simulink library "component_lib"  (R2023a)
settings: Solver=VariableStepAuto  StartTime=0.0  StopTime=10.0  RelTol=1e-3
undefined symbols (not defined in the file or in its folder): component_lib, ECCV_r, KoblenzTrier, mm, par, param_TD04, R1234yf_ph, SigIdentifier, Systems, TH0023_WP120, Thermal, V_nom
libraries: base_lib x166, $bdroot x164, simulink x2, slpidlib x1
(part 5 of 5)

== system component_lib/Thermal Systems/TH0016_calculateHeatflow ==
  "CL: (T1, p1, W1)" : Inport
  "CL: (T2, p2, W2)" : Inport  Port=2
  Constant2 : Constant  Value=par.cp_clt
  Demux : Demux  Outputs=3
  Demux1 : Demux  Outputs=3
  Product : Product  Inputs=3
  Sum : Sum  Inputs=|-+
  Terminator : Terminator
  Terminator1 : Terminator
  Terminator2 : Terminator
  Q [J/s] : Outport
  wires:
  "CL: (T1, p1, W1)"/1 -> Demux/1
  "CL: (T2, p2, W2)"/1 -> Demux1/1
  Constant2/1 -> Product/2
  Product/1 -> Q [J/s]/1
  Demux/2 -> Terminator/1
  Demux1/2 -> Terminator1/1
  Demux1/3 -> Terminator2/1
  Demux1/1 -> Sum/2
  Sum/1 -> Product/1
  Demux/1 -> Sum/1
  Demux/3 -> Product/3

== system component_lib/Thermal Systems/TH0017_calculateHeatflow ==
  "AIR: (T1, p1, W1)" : Inport
  "AIR: (T2, p2, W2)" : Inport  Port=2
  Constant2 : Constant  Value=par.cp_air
  Demux : Demux  Outputs=3
  Demux1 : Demux  Outputs=3
  Product : Product  Inputs=3
  Sum : Sum  Inputs=|-+
  Terminator : Terminator
  Terminator1 : Terminator
  Terminator2 : Terminator
  Q [J/s] : Outport
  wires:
  "AIR: (T1, p1, W1)"/1 -> Demux/1
  "AIR: (T2, p2, W2)"/1 -> Demux1/1
  Constant2/1 -> Product/2
  Product/1 -> Q [J/s]/1
  Demux/2 -> Terminator/1
  Demux1/2 -> Terminator1/1
  Demux1/3 -> Terminator2/1
  Demux1/1 -> Sum/2
  Sum/1 -> Product/1
  Demux/1 -> Sum/1
  Demux/3 -> Product/3

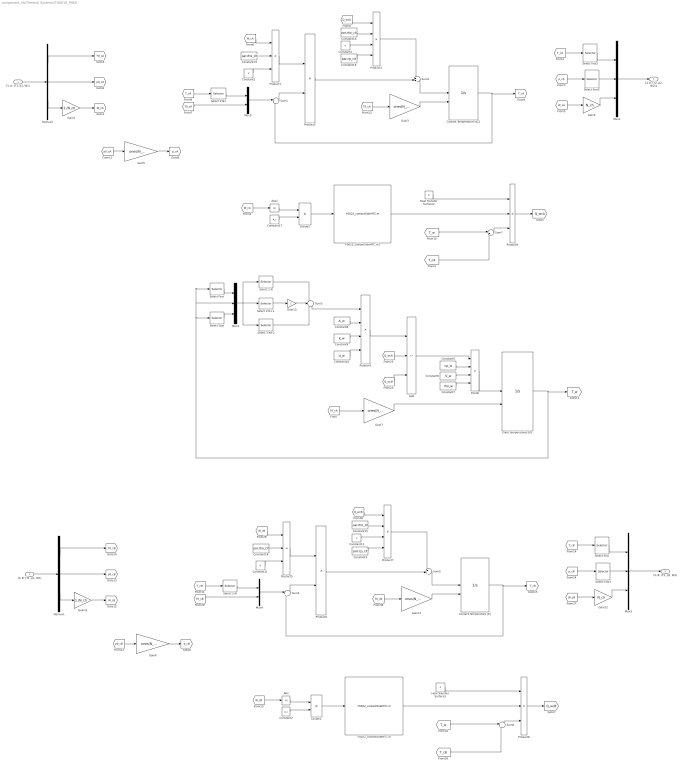
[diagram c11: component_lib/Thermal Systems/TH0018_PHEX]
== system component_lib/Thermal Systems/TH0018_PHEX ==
  "CL A: (T1, p1, W1)" : Inport
  "CL B: (T1, p1, W1)" : Inport  Port=2
  Abs : Abs
  Abs1 : Abs
  Add : Sum  Inputs=+--
  Constant{1,4,11..12} (4 alike) : Constant  Value=V
  Constant10 : Constant  Value=d_w
  Constant{13..16} (4 alike) : Constant  Value=par.rho_clt
  Constant17 : Constant  Value=A_c
  Constant18 : Constant  Value=par.cp_clt
  Constant2 : Constant  Value=A_c
  Constant3 : Constant  Value=par.cp_clt
  Constant5 : Constant  Value=cp_w
  Constant6 : Constant  Value=V_w
  Constant7 : Constant  Value=rho_w
  Constant8 : Constant  Value=A_w
  Constant9 : Constant  Value=k_w
  Coolant Temperature [K] : Integrator  InitialConditionSource=external  LimitOutput=on  LowerSaturationLimit=0
  Coolant Temperature [K]1 : Integrator  InitialConditionSource=external  LimitOutput=on  LowerSaturationLimit=0
  Demux1 : Demux  Outputs=3
  Demux2 : Demux  Outputs=3
  Divide : Product  Inputs=*///
  Divide1 : Product  Inputs=*/
  Divide2 : Product  Inputs=*/
  F0022_coolantSideHTC.m : base_lib/F0022_heatPump/F0022_coolantSideHTC.m  SystemSampleTime=-1  VariantActivationTime=update diagram  Latency=0  AutoFrameSizeCalculation=off
  F0022_coolantSideHTC.m1 : base_lib/F0022_heatPump/F0022_coolantSideHTC.m  SystemSampleTime=-1  VariantActivationTime=update diagram  Latency=0  AutoFrameSizeCalculation=off
  Gain1 : Gain  Gain=1./N_ch
  Gain10 : Gain  Gain=2
  Gain11 : Gain  Gain=1./N_ch
  Gain12 : Gain  Gain=N_ch
  Gain{3..5,7,13} (5 alike) : Gain  Gain=ones(N_nod,1)
  Gain2 : Gain  Gain=N_ch
  Heat Transfer Surface1 : Constant  Value=A
  Heat Transfer Surface2 : Constant  Value=A
  Mux1 : Mux  Inputs=3
  Mux2 : Mux  Inputs=3
  Mux3 : Mux  Inputs=3
  Mux4 : Mux  Inputs=2
  Mux5 : Mux  Inputs=2
  Plate temperatures [K] : Integrator  InitialConditionSource=external  LimitOutput=on  LowerSaturationLimit=0
  Product1 : Product  Inputs=*//
  Product2 : Product
  Product3 : Product  Inputs=*///
  Product4 : Product  Inputs=***/
  Product5 : Product  Inputs=*//
  Product6 : Product
  Product7 : Product  Inputs=*///
  Product8 : Product  Inputs=3
  Product9 : Product  Inputs=3
  Select 1:N : Selector  InputPortWidth=N_nod+2  IndexOptions=Index vector (dialog)  Indices=[1:N_nod]  OutputSizes=1
  Select 2:N : Selector  InputPortWidth=N_nod  IndexOptions=Index vector (dialog)  Indices=[2:N_nod]  OutputSizes=1
  "Select 2:N+1 " : Selector  InputPortWidth=N_nod+2  IndexOptions=Index vector (dialog)  Indices=[2:(N_nod+1)]  OutputSizes=1
  Select 2:N1 : Selector  InputPortWidth=N_nod  IndexOptions=Index vector (dialog)  Indices=[2:N_nod]  OutputSizes=1
  Select 3:N+2 : Selector  InputPortWidth=N_nod+2  IndexOptions=Index vector (dialog)  Indices=[3:(N_nod+2)]  OutputSizes=1
  Select First : Selector  InputPortWidth=N_nod  IndexOptions=Index vector (dialog)  Indices=1  OutputSizes=1
  Select Last : Selector  InputPortWidth=N_nod  IndexOptions=Index vector (dialog)  Indices=N_nod  OutputSizes=1
  Select first{,1..3} (4 alike) : Selector  InputPortWidth=N_nod  IndexOptions=Index vector (dialog)  Indices=1  OutputSizes=1
  Sum{1,4,6..7} (4 alike) : Sum  Inputs=|+-
  Sum2 : Sum  Inputs=++|
  Sum3 : Sum  Inputs=+-+
  Sum5 : Sum  Inputs=++|
  "CL A: (T2, p2, W2)1" : Outport
  "CL B: (T2, p2, W2)" : Outport  Port=2
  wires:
  Gain7/1 -> Plate temperatures [K]/2
  Divide/1 -> Plate temperatures [K]/1
  Add/1 -> Divide/1
  Constant5/1 -> Divide/2
  Constant6/1 -> Divide/3
  Constant7/1 -> Divide/4
  [Q_wcB] -> Add/3
  Plate temperatures [K]/1 -> [T_w], Select First/1, Mux2/2, Select Last/1
  Select First/1 -> Mux2/1
  Mux2/1 -> Select 3:N+2/1, "Select 2:N+1 "/1, Select 1:N/1
  Select Last/1 -> Mux2/3
  "Select 2:N+1 "/1 -> Gain10/1
  Gain10/1 -> Sum3/2
  Select 1:N/1 -> Sum3/1
  Select 3:N+2/1 -> Sum3/3
  Sum3/1 -> Product4/1
  Constant8/1 -> Product4/2
  Constant9/1 -> Product4/3
  Constant10/1 -> Product4/4
  Product4/1 -> Add/1
  [Q_wcA] -> Add/2
  Gain11/1 -> [W_cB]
  Demux1/2 -> [p0_cB]
  "CL B: (T1, p1, W1)"/1 -> Demux1/1
  [T_cB] -> Select first/1
  Select first1/1 -> Mux3/2
  [W_cB] -> Gain12/1
  Mux3/1 -> "CL B: (T2, p2, W2)"/1
  [p_cB] -> Select first1/1
  [Q_wcB] -> Product7/1
  Mux4/1 -> Sum4/1
  Coolant Temperature [K]/1 -> [T_cB], Sum4/2
  Product7/1 -> Sum5/1
  Gain13/1 -> Coolant Temperature [K]/2
  [T_cB] -> Select 2:N/1
  Sum5/1 -> Coolant Temperature [K]/1
  Sum4/1 -> Product6/2
  Constant15/1 -> Product7/2
  Product5/1 -> Product6/1
  [W_cB] -> Product5/1
  Product6/1 -> Sum5/2
  Constant3/1 -> Product7/4
  Constant14/1 -> Product5/2
  Divide1/1 -> F0022_coolantSideHTC.m/1
  Product8/1 -> [Q_wcB]
  F0022_coolantSideHTC.m/1 -> Product8/2
  Sum6/1 -> Product8/3
  [T_cB] -> Sum6/2
  Gain4/1 -> [p_cB]
  [p0_cB] -> Gain4/1
  [T_w] -> Sum6/1
  Heat Transfer Surface1/1 -> Product8/1
  Constant11/1 -> Product5/3
  Constant12/1 -> Product7/3
  [T0_cB] -> Mux4/2
  Select 2:N/1 -> Mux4/1
  Gain12/1 -> Mux3/3
  Select first/1 -> Mux3/1
  Demux1/3 -> Gain11/1
  Demux1/1 -> [T0_cB]
  [T0_cA] -> Gain7/1
  [T0_cB] -> Gain13/1
  Abs/1 -> Divide1/1
  Constant2/1 -> Divide1/2
  [W_cB] -> Abs/1
  [T_cA] -> Sum7/2
  Gain2/1 -> Mux1/3
  Constant13/1 -> Product1/2
  Select 2:N1/1 -> Mux5/1
  Select first2/1 -> Mux1/1
  Demux2/2 -> [p0_cA]
  Divide2/1 -> F0022_coolantSideHTC.m1/1
  [T_cA] -> Select first2/1
  Constant1/1 -> Product1/3
  [W_cA] -> Product1/1
  Gain5/1 -> [p_cA]
  Sum7/1 -> Product9/3
  Demux2/3 -> Gain1/1
  Constant18/1 -> Product3/4
  [Q_wcA] -> Product3/1
  F0022_coolantSideHTC.m1/1 -> Product9/2
  [T0_cA] -> Mux5/2
  [W_cA] -> Abs1/1
  Constant17/1 -> Divide2/2
  Sum2/1 -> Coolant Temperature [K]1/1
  Constant16/1 -> Product3/2
  Demux2/1 -> [T0_cA]
  [T0_cA] -> Gain3/1
  Gain1/1 -> [W_cA]
  Sum1/1 -> Product2/2
  [T_cA] -> Select 2:N1/1
  Product3/1 -> Sum2/1
  Gain3/1 -> Coolant Temperature [K]1/2
  [p_cA] -> Select first3/1
  Mux5/1 -> Sum1/1
  Coolant Temperature [K]1/1 -> [T_cA], Sum1/2
  Constant4/1 -> Product3/3
  Product2/1 -> Sum2/2
  Product9/1 -> [Q_wcA]
  [T_w] -> Sum7/1
  Mux1/1 -> "CL A: (T2, p2, W2)1"/1
  Product1/1 -> Product2/1
  Select first3/1 -> Mux1/2
  [p0_cA] -> Gain5/1
  "CL A: (T1, p1, W1)"/1 -> Demux2/1
  Heat Transfer Surface2/1 -> Product9/1
  [W_cA] -> Gain2/1
  Abs1/1 -> Divide2/1

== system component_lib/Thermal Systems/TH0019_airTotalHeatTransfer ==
  Q [J/s] : Inport
  AIR: (T1,p1,W1) : Inport  Port=2
  Constant : Constant  Value=par.cp_air
  Demux : Demux  Outputs=3
  Mux : Mux  Inputs=3
  Product : Product  Inputs=*//
  Sum : Sum  Inputs=++|
  AIR: (T2,p2,W2) : Outport
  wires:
  AIR: (T1,p1,W1)/1 -> Demux/1
  Mux/1 -> AIR: (T2,p2,W2)/1
  Demux/3 -> Mux/3, Product/2
  Demux/2 -> Mux/2
  Sum/1 -> Mux/1
  Q [J/s]/1 -> Product/1
  Constant/1 -> Product/3
  Demux/1 -> Sum/2
  Product/1 -> Sum/1

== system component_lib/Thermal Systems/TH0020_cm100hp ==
  V_sup [V] : Inport
  V_ctrl [V] : Inport  Port=2
  CL: (T1,p1,W1) : Inport  Port=3
  Constant : Constant  Value=par.rho_clt
  Constant5 : Constant  Value=27.5
  Demux : Demux  Outputs=3
  Divide : Product  Inputs=/*
  Divide1 : Product  Inputs=*/
  Divide2 : Product  Inputs=*/
  F0023_current.m : base_lib/F0023_epirocWaterPump/F0023_current.m  SystemSampleTime=-1  VariantActivationTime=update diagram  Latency=0  AutoFrameSizeCalculation=off
  F0023_pressure.m : base_lib/F0023_epirocWaterPump/F0023_pressure.m  SystemSampleTime=-1  VariantActivationTime=update diagram  Latency=0  AutoFrameSizeCalculation=off
  F0023_speed.m : base_lib/F0023_epirocWaterPump/F0023_speed.m  SystemSampleTime=-1  VariantActivationTime=update diagram  Latency=0  AutoFrameSizeCalculation=off
  Gain : Gain  Gain=1e5
  Gain1 : Gain
  Integrator Limited : Integrator  InitialConditionSource=external  LimitOutput=on  UpperSaturationLimit=10  LowerSaturationLimit=0
  Mux : Mux  Inputs=3
  Product : Product
  Product1 : Product  Inputs=3
  Sum : Sum  Inputs=|++
  Sum1 : Sum  Inputs=-|+
  Terminator : Terminator
  I [A] : Outport
  P_hydr [J/s] : Outport  Port=2
  CL: (T2,p2,W2) : Outport  Port=3
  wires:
  CL: (T1,p1,W1)/1 -> Demux/1
  Mux/1 -> CL: (T2,p2,W2)/1
  Integrator Limited/1 -> F0023_speed.m/2, F0023_current.m/2, Sum1/1, F0023_pressure.m/2
  Demux/2 -> Sum/1
  Sum/1 -> Mux/2
  Demux/3 -> [q], F0023_speed.m/1, F0023_current.m/1, F0023_pressure.m/1, Mux/3
  Demux/1 -> Mux/1
  F0023_pressure.m/1 -> Gain/1
  Sum1/1 -> Gain1/1
  V_ctrl [V]/1 -> Sum1/2, Integrator Limited/2
  Gain1/1 -> Integrator Limited/1
  V_sup [V]/1 -> Divide1/2, [V_sup]
  Divide1/1 -> I [A]/1
  Product/1 -> P_hydr [J/s]/1
  Constant/1 -> Divide2/2
  Divide2/1 -> Product/2
  [q] -> Divide2/1
  [V_sup] -> Divide/1, Product1/1
  F0023_current.m/1 -> Product1/3
  Divide/1 -> Product1/2
  Constant5/1 -> Divide/2
  Product1/1 -> Divide1/1
  F0023_speed.m/1 -> Terminator/1
  Gain/1 -> Product/1, Sum/2

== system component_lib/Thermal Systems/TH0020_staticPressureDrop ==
  CL: (T1,p1,W1) : Inport
  Constant : Constant  Value=dp
  Demux : Demux  Outputs=3
  Mux : Mux  Inputs=3
  Sum : Sum  Inputs=|+-
  CL: (T2,p2,W2) : Outport
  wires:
  CL: (T1,p1,W1)/1 -> Demux/1
  Mux/1 -> CL: (T2,p2,W2)/1
  Demux/2 -> Sum/1
  Sum/1 -> Mux/2
  Demux/3 -> Mux/3
  Demux/1 -> Mux/1
  Constant/1 -> Sum/2

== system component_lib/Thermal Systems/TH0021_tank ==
  p [Pa] : Inport
  CL: (T1,p1,W1) : Inport  Port=2
  Constant : Constant  Value=par.cv_clt
  Constant2 : Constant  Value=T0
  Constant3 : Constant  Value=V .* par.rho_clt
  Demux1 : Demux  Outputs=3
  Divide : Product  Inputs=*//
  F0017_temperatureToEnthalpy.m : base_lib/F0017_channelCooling/F0017_temperatureToEnthalpy.m  SystemSampleTime=-1  VariantActivationTime=update diagram  Latency=0  AutoFrameSizeCalculation=off
  F0017_temperatureToEnthalpy.m1 : base_lib/F0017_channelCooling/F0017_temperatureToEnthalpy.m  SystemSampleTime=-1  VariantActivationTime=update diagram  Latency=0  AutoFrameSizeCalculation=off
  Gain : Gain  Gain=1e-3
  Integrator : Integrator  InitialCondition=1  LimitOutput=on  LowerSaturationLimit=0
  Integrator2 : Integrator  InitialConditionSource=external  InitialCondition=293  LimitOutput=on  LowerSaturationLimit=1e-3
  Mux1 : Mux  Inputs=3
  Product : Product
  Product1 : Product
  Sum : Sum  Inputs=-+|
  Sum2 : Sum  Inputs=+|-
  W [kg/s] : Outport
  CL: (T2,p2,W2) : Outport  Port=2
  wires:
  Product/1 -> Sum2/1
  Sum2/1 -> Divide/1
  Constant2/1 -> Integrator2/2
  Demux1/1 -> F0017_temperatureToEnthalpy.m/1
  Integrator2/1 -> [T], Mux1/1
  Constant/1 -> Divide/2
  Mux1/1 -> CL: (T2,p2,W2)/1
  F0017_temperatureToEnthalpy.m1/1 -> Product1/1
  F0017_temperatureToEnthalpy.m/1 -> Product/1
  Divide/1 -> Integrator2/1
  CL: (T1,p1,W1)/1 -> Demux1/1
  Demux1/3 -> Product/2
  p [Pa]/1 -> Sum/1, Mux1/2
  Demux1/2 -> [p1]
  Constant3/1 -> Divide/3
  Product1/1 -> Sum2/2
  Gain/1 -> Integrator/1
  [p1] -> Sum/2
  Integrator/1 -> Product1/2, W [kg/s]/1, Mux1/3
  Sum/1 -> Gain/1
  [T] -> F0017_temperatureToEnthalpy.m1/1

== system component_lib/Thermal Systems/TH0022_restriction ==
  CL: (T1,p1,W1) : Inport
  Demux : Demux  Outputs=3
  F0017_restriction.m : base_lib/F0017_channelCooling/F0017_restriction.m  SystemSampleTime=-1  VariantActivationTime=update diagram  Latency=0  AutoFrameSizeCalculation=off
  Mux : Mux  Inputs=3
  Sum : Sum  Inputs=|+-
  CL: (T2,p2,W2) : Outport
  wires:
  CL: (T1,p1,W1)/1 -> Demux/1
  Mux/1 -> CL: (T2,p2,W2)/1
  Demux/3 -> Mux/3, F0017_restriction.m/1
  Demux/2 -> Sum/1
  Sum/1 -> Mux/2
  F0017_restriction.m/1 -> Sum/2
  Demux/1 -> Mux/1

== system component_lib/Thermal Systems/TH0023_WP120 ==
  V_sup [V] : Inport
  n [rpm] : Inport  Port=2
  CL: (T1,p1,W1) : Inport  Port=3
  Constant : Constant  Value=par.rho_clt
  Demux : Demux  Outputs=3
  Divide : Product  Inputs=*/
  Divide2 : Product  Inputs=*/
  F0024_powerWP120.m : base_lib/F0024_WPpumps/F0024_powerWP120.m  SystemSampleTime=-1  VariantActivationTime=update diagram  Latency=0  AutoFrameSizeCalculation=off
  F0024_pressureWP120.m : base_lib/F0024_WPpumps/F0024_pressureWP120.m  SystemSampleTime=-1  VariantActivationTime=update diagram  Latency=0  AutoFrameSizeCalculation=off
  Gain1 : Gain
  Integrator Limited : Integrator  InitialConditionSource=external  LimitOutput=on  UpperSaturationLimit=6000  LowerSaturationLimit=0
  Mux : Mux  Inputs=3
  Product : Product
  Sum : Sum  Inputs=|++
  Sum1 : Sum  Inputs=-|+
  I [A] : Outport
  P_hydr [J/s] : Outport  Port=2
  CL: (T2,p2,W2) : Outport  Port=3
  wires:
  F0024_pressureWP120.m/1 -> Sum/2, Product/1
  F0024_powerWP120.m/1 -> Divide/1
  [q] -> Divide2/1
  Divide2/1 -> Product/2
  Constant/1 -> Divide2/2
  Product/1 -> P_hydr [J/s]/1
  Gain1/1 -> Integrator Limited/1
  n [rpm]/1 -> Integrator Limited/2, Sum1/2
  Sum1/1 -> Gain1/1
  Demux/1 -> Mux/1
  Demux/3 -> Mux/3, F0024_powerWP120.m/1, F0024_pressureWP120.m/1, [q]
  Sum/1 -> Mux/2
  Demux/2 -> Sum/1
  Integrator Limited/1 -> F0024_powerWP120.m/2, F0024_pressureWP120.m/2, Sum1/1
  Mux/1 -> CL: (T2,p2,W2)/1
  CL: (T1,p1,W1)/1 -> Demux/1
  Divide/1 -> I [A]/1
  V_sup [V]/1 -> Divide/2

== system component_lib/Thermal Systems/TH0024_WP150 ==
  V_sup [V] : Inport
  n [rpm] : Inport  Port=2
  CL: (T1,p1,W1) : Inport  Port=3
  Constant : Constant  Value=par.rho_clt
  Demux : Demux  Outputs=3
  Divide : Product  Inputs=*/
  Divide2 : Product  Inputs=*/
  F0024_powerWP150.m : base_lib/F0024_WPpumps/F0024_powerWP150.m  SystemSampleTime=-1  VariantActivationTime=update diagram  Latency=0  AutoFrameSizeCalculation=off
  F0024_pressureWP150.m : base_lib/F0024_WPpumps/F0024_pressureWP150.m  SystemSampleTime=-1  VariantActivationTime=update diagram  Latency=0  AutoFrameSizeCalculation=off
  Gain1 : Gain
  Integrator Limited : Integrator  InitialConditionSource=external  LimitOutput=on  UpperSaturationLimit=4500  LowerSaturationLimit=0
  Mux : Mux  Inputs=3
  Product : Product
  Sum : Sum  Inputs=|++
  Sum1 : Sum  Inputs=-|+
  I [A] : Outport
  P_hydr [J/s] : Outport  Port=2
  CL: (T2,p2,W2) : Outport  Port=3
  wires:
  F0024_pressureWP150.m/1 -> Sum/2, Product/1
  F0024_powerWP150.m/1 -> Divide/1
  [q] -> Divide2/1
  Divide2/1 -> Product/2
  Constant/1 -> Divide2/2
  Product/1 -> P_hydr [J/s]/1
  Gain1/1 -> Integrator Limited/1
  n [rpm]/1 -> Integrator Limited/2, Sum1/2
  Sum1/1 -> Gain1/1
  Demux/1 -> Mux/1
  Demux/3 -> Mux/3, F0024_powerWP150.m/1, F0024_pressureWP150.m/1, [q]
  Sum/1 -> Mux/2
  Demux/2 -> Sum/1
  Integrator Limited/1 -> F0024_powerWP150.m/2, F0024_pressureWP150.m/2, Sum1/1
  Mux/1 -> CL: (T2,p2,W2)/1
  CL: (T1,p1,W1)/1 -> Demux/1
  Divide/1 -> I [A]/1
  V_sup [V]/1 -> Divide/2

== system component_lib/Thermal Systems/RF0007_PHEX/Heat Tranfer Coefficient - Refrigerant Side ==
  W_r [kg/s] : Inport
  x_r [-] : Inport  Port=2
  T_r [K] : Inport  Port=3
  Constant : Constant  Value=A_c
  Constant1 : Constant  Value=1.5 .* par.Tc
  Constant3 : Constant  Value=1.5 .* par.Tc
  Divide : Product  Inputs=*/
  F0021_cp.m : base_lib/F0021_R1234yf/F0021_cp.m  SystemSampleTime=-1  VariantActivationTime=update diagram  Latency=0  AutoFrameSizeCalculation=off
  F0021_cp.m1 : base_lib/F0021_R1234yf/F0021_cp.m  SystemSampleTime=-1  VariantActivationTime=update diagram  Latency=0  AutoFrameSizeCalculation=off
  F0021_cv.m : base_lib/F0021_R1234yf/F0021_cv.m  SystemSampleTime=-1  VariantActivationTime=update diagram  Latency=0  AutoFrameSizeCalculation=off
  F0021_cv.m1 : base_lib/F0021_R1234yf/F0021_cv.m  SystemSampleTime=-1  VariantActivationTime=update diagram  Latency=0  AutoFrameSizeCalculation=off
  F0021_dliqsat.m : base_lib/F0021_R1234yf/F0021_dliqsat.m  SystemSampleTime=-1  VariantActivationTime=update diagram  Latency=0  AutoFrameSizeCalculation=off
  F0021_dpdrho.m{,1..3} (4 alike) : base_lib/F0021_R1234yf/F0021_dpdrho.m  SystemSampleTime=-1  VariantActivationTime=update diagram  Latency=0  AutoFrameSizeCalculation=off
  F0021_dvapsat.m : base_lib/F0021_R1234yf/F0021_dvapsat.m  SystemSampleTime=-1  VariantActivationTime=update diagram  Latency=0  AutoFrameSizeCalculation=off
  F0022_OSFPHEX.m : base_lib/F0022_heatPump/F0022_OSFPHEX.m  SystemSampleTime=-1  VariantActivationTime=update diagram  Latency=0  AutoFrameSizeCalculation=off
  Gain1 : Gain  Gain=1/par.M
  Gain4 : Gain  Gain=1/par.M
  Gain7 : Gain  Gain=par.M
  Gain9 : Gain  Gain=par.M
  R1234yf_lambda.m : base_lib/F0021_R1234yf/R1234yf_lambda.m  SystemSampleTime=-1  VariantActivationTime=update diagram  Latency=0  AutoFrameSizeCalculation=off
  R1234yf_lambda.m1 : base_lib/F0021_R1234yf/R1234yf_lambda.m  SystemSampleTime=-1  VariantActivationTime=update diagram  Latency=0  AutoFrameSizeCalculation=off
  R1234yf_mu.m : base_lib/F0021_R1234yf/R1234yf_mu.m  SystemSampleTime=-1  VariantActivationTime=update diagram  Latency=0  AutoFrameSizeCalculation=off
  R1234yf_mu.m1 : base_lib/F0021_R1234yf/R1234yf_mu.m  SystemSampleTime=-1  VariantActivationTime=update diagram  Latency=0  AutoFrameSizeCalculation=off
  R1234yf_sigma.m : base_lib/F0021_R1234yf/R1234yf_sigma.m  SystemSampleTime=-1  VariantActivationTime=update diagram  Latency=0  AutoFrameSizeCalculation=off
  h [W/mK] : Outport
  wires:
  [cp_f] -> R1234yf_lambda.m/3
  Divide/1 -> F0022_OSFPHEX.m/1
  F0021_dpdrho.m1/1 -> R1234yf_lambda.m/7
  F0021_dliqsat.m/1 -> F0021_dpdrho.m1/2, F0021_dpdrho.m/2, F0021_cv.m/2, R1234yf_lambda.m/2, R1234yf_mu.m/2, F0021_cp.m/2, Gain9/1
  F0021_cv.m/1 -> R1234yf_lambda.m/4
  Constant3/1 -> F0021_dpdrho.m1/1
  R1234yf_mu.m/1 -> F0022_OSFPHEX.m/7, [mu_f]
  x_r [-]/1 -> F0022_OSFPHEX.m/2
  F0021_dpdrho.m/1 -> R1234yf_lambda.m/6
  R1234yf_sigma.m/1 -> F0022_OSFPHEX.m/11
  F0021_dvapsat.m/1 -> R1234yf_lambda.m1/2, F0021_dpdrho.m3/2, F0021_dpdrho.m2/2, F0021_cv.m1/2, R1234yf_mu.m1/2, F0021_cp.m1/2, Gain7/1
  Gain7/1 -> F0022_OSFPHEX.m/4
  R1234yf_lambda.m/1 -> F0022_OSFPHEX.m/9
  [mu_f] -> R1234yf_lambda.m/5
  W_r [kg/s]/1 -> Divide/1
  Gain4/1 -> F0022_OSFPHEX.m/5
  Gain9/1 -> F0022_OSFPHEX.m/3
  F0021_cp.m/1 -> [cp_f], Gain4/1
  F0022_OSFPHEX.m/1 -> h [W/mK]/1
  Gain1/1 -> F0022_OSFPHEX.m/6
  F0021_cp.m1/1 -> [cp_g], Gain1/1
  R1234yf_mu.m1/1 -> [mu_g], F0022_OSFPHEX.m/8
  [mu_g] -> R1234yf_lambda.m1/5
  Constant1/1 -> F0021_dpdrho.m3/1
  T_r [K]/1 -> F0021_cp.m1/1, R1234yf_mu.m1/1, F0021_dpdrho.m2/1, F0021_cv.m1/1, R1234yf_lambda.m1/1, F0021_dpdrho.m/1, F0021_cv.m/1, R1234yf_lambda.m/1, R1234yf_sigma.m/1, R1234yf_mu.m/1, F0021_cp.m/1, F0021_dvapsat.m/1, F0021_dliqsat.m/1
  F0021_dpdrho.m3/1 -> R1234yf_lambda.m1/7
  F0021_cv.m1/1 -> R1234yf_lambda.m1/4
  F0021_dpdrho.m2/1 -> R1234yf_lambda.m1/6
  [cp_g] -> R1234yf_lambda.m1/3
  R1234yf_lambda.m1/1 -> F0022_OSFPHEX.m/10
  Constant/1 -> Divide/2

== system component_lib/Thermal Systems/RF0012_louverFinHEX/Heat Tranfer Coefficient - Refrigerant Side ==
  W_r [kg/s] : Inport
  x_r [-] : Inport  Port=2
  T_r [K] : Inport  Port=3
  Abs : Abs
  Constant1 : Constant  Value=1.5 .* par.Tc
  Constant3 : Constant  Value=1.5 .* par.Tc
  F0021_cp.m : base_lib/F0021_R1234yf/F0021_cp.m  SystemSampleTime=-1  VariantActivationTime=update diagram  Latency=0  AutoFrameSizeCalculation=off
  F0021_cp.m1 : base_lib/F0021_R1234yf/F0021_cp.m  SystemSampleTime=-1  VariantActivationTime=update diagram  Latency=0  AutoFrameSizeCalculation=off
  F0021_cv.m : base_lib/F0021_R1234yf/F0021_cv.m  SystemSampleTime=-1  VariantActivationTime=update diagram  Latency=0  AutoFrameSizeCalculation=off
  F0021_cv.m1 : base_lib/F0021_R1234yf/F0021_cv.m  SystemSampleTime=-1  VariantActivationTime=update diagram  Latency=0  AutoFrameSizeCalculation=off
  F0021_dliqsat.m : base_lib/F0021_R1234yf/F0021_dliqsat.m  SystemSampleTime=-1  VariantActivationTime=update diagram  Latency=0  AutoFrameSizeCalculation=off
  F0021_dpdrho.m{,1..3} (4 alike) : base_lib/F0021_R1234yf/F0021_dpdrho.m  SystemSampleTime=-1  VariantActivationTime=update diagram  Latency=0  AutoFrameSizeCalculation=off
  F0021_dvapsat.m : base_lib/F0021_R1234yf/F0021_dvapsat.m  SystemSampleTime=-1  VariantActivationTime=update diagram  Latency=0  AutoFrameSizeCalculation=off
  F0021_psat.m : base_lib/F0021_R1234yf/F0021_psat.m  SystemSampleTime=-1  VariantActivationTime=update diagram  Latency=0  AutoFrameSizeCalculation=off
  F0022_massFlux.m : base_lib/F0022_heatPump/F0022_massFlux.m  SystemSampleTime=-1  VariantActivationTime=update diagram  Latency=0  AutoFrameSizeCalculation=off
  F0022_minichannelCondensingHTC.m : base_lib/F0022_heatPump/F0022_minichannelCondensingHTC.m  SystemSampleTime=-1  VariantActivationTime=update diagram  Latency=0  AutoFrameSizeCalculation=off
  Gain1 : Gain  Gain=1/par.M
  Gain4 : Gain  Gain=1/par.M
  Gain7 : Gain  Gain=par.M
  Gain9 : Gain  Gain=par.M
  R1234yf_lambda.m : base_lib/F0021_R1234yf/R1234yf_lambda.m  SystemSampleTime=-1  VariantActivationTime=update diagram  Latency=0  AutoFrameSizeCalculation=off
  R1234yf_lambda.m1 : base_lib/F0021_R1234yf/R1234yf_lambda.m  SystemSampleTime=-1  VariantActivationTime=update diagram  Latency=0  AutoFrameSizeCalculation=off
  R1234yf_mu.m : base_lib/F0021_R1234yf/R1234yf_mu.m  SystemSampleTime=-1  VariantActivationTime=update diagram  Latency=0  AutoFrameSizeCalculation=off
  R1234yf_mu.m1 : base_lib/F0021_R1234yf/R1234yf_mu.m  SystemSampleTime=-1  VariantActivationTime=update diagram  Latency=0  AutoFrameSizeCalculation=off
  h [W/mK] : Outport
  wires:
  F0022_minichannelCondensingHTC.m/1 -> h [W/mK]/1
  W_r [kg/s]/1 -> Abs/1
  F0021_cp.m/1 -> [cp_f], Gain4/1
  Gain9/1 -> F0022_minichannelCondensingHTC.m/4
  Gain4/1 -> F0022_minichannelCondensingHTC.m/6
  Abs/1 -> F0022_massFlux.m/1
  [mu_f] -> R1234yf_lambda.m/5
  F0021_dvapsat.m/1 -> [rho_g], Gain7/1, F0021_cp.m1/2, R1234yf_mu.m1/2
  F0021_dpdrho.m/1 -> R1234yf_lambda.m/6
  R1234yf_mu.m/1 -> F0022_minichannelCondensingHTC.m/8, [mu_f]
  Constant3/1 -> F0021_dpdrho.m1/1
  F0021_cv.m/1 -> R1234yf_lambda.m/4
  F0021_dliqsat.m/1 -> R1234yf_mu.m/2, F0021_cp.m/2, [rho_f], Gain9/1
  F0021_dpdrho.m1/1 -> R1234yf_lambda.m/7
  F0022_massFlux.m/1 -> F0022_minichannelCondensingHTC.m/1
  [cp_f] -> R1234yf_lambda.m/3
  Gain7/1 -> F0022_minichannelCondensingHTC.m/5
  [rho_f] -> F0021_dpdrho.m1/2, F0021_dpdrho.m/2, F0021_cv.m/2, R1234yf_lambda.m/2
  F0021_psat.m/1 -> F0022_minichannelCondensingHTC.m/2
  F0021_cp.m1/1 -> [cp_g], Gain1/1
  Gain1/1 -> F0022_minichannelCondensingHTC.m/7
  R1234yf_mu.m1/1 -> [mu_g], F0022_minichannelCondensingHTC.m/9
  [rho_g] -> F0021_dpdrho.m3/2, F0021_dpdrho.m2/2, F0021_cv.m1/2, R1234yf_lambda.m1/2
  [cp_g] -> R1234yf_lambda.m1/3
  F0021_dpdrho.m3/1 -> R1234yf_lambda.m1/7
  Constant1/1 -> F0021_dpdrho.m3/1
  [mu_g] -> R1234yf_lambda.m1/5
  T_r [K]/1 -> F0021_cp.m1/1, R1234yf_mu.m/1, F0021_dpdrho.m2/1, F0021_cv.m1/1, R1234yf_lambda.m1/1, F0021_dpdrho.m/1, F0021_cv.m/1, R1234yf_lambda.m/1, R1234yf_mu.m1/1, F0021_cp.m/1, F0021_dvapsat.m/1, F0021_dliqsat.m/1, F0021_psat.m/1
  F0021_dpdrho.m2/1 -> R1234yf_lambda.m1/6
  F0021_cv.m1/1 -> R1234yf_lambda.m1/4
  R1234yf_lambda.m1/1 -> F0022_minichannelCondensingHTC.m/11
  R1234yf_lambda.m/1 -> F0022_minichannelCondensingHTC.m/10
  x_r [-]/1 -> F0022_minichannelCondensingHTC.m/3
